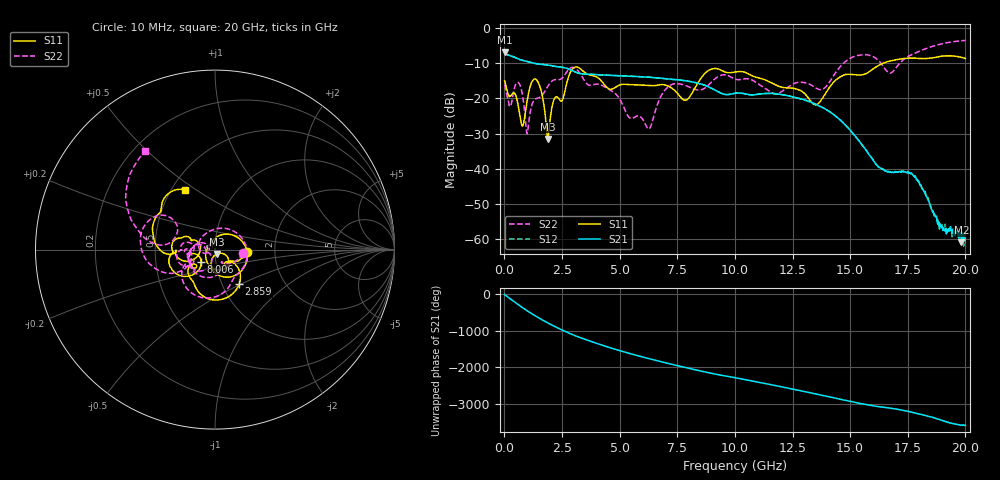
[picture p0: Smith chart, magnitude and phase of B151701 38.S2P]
!  2-Port S-parameters saved by WinCal
! VAR MeasName=S-Parameters (CALIBRATED_DATA) read from VNA (N5244A)
! VAR MeasDate=2015-12-24 19:13:49
! VAR NAME=B151701 38
! VAR FILENAME=B151701 38.S2P
! VAR DATE=2015-12-24 19:13:49
! VAR PHYS_PORTS=1,3
# Hz S DB R 50
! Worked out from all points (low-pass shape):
!   801 points, 10 MHz to 20 GHz, reference 50 ohm
!   highest |S21| = -6.86 dB at 10 MHz (marker M1); lowest = -61.0 dB at 19.83 GHz (marker M2)
!   |S21| within 3 dB of the highest: start of sweep to 1.204 GHz
!   lowest |S11| = -31.5 dB at 1.884 GHz (marker M3), VSWR 1.05, Z = 51 - j2.5 ohm
!   |S11| at or under -10 dB: start of sweep to 16.41 GHz
!   |S22| runs from -30.0 to -3.5 dB; largest |S21 - S12| = 0.0011
!   S11 on the Smith chart (normalised r, x): 10 MHz: 1.43, -0.04; 2.859 GHz: 1.20, -0.49; 8.006 GHz: 0.85, -0.12; 20 GHz: 0.59, +0.45
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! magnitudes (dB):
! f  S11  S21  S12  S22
! 10 MHz  -15.0  -6.9  -6.8  -16.1
! 234.9 MHz  -19.1  -7.8  -7.8  -22.0
! 534.7 MHz  -20.0  -8.5  -8.5  -15.5
! 759.6 MHz  -27.7  -9.1  -9.1  -18.1
! 1.01 GHz  -19.9  -9.5  -9.5  -29.5
! 1.434 GHz  -15.0  -10.1  -10.1  -19.9
! 1.884 GHz  -31.5  -10.5  -10.4  -16.5
! 2.159 GHz  -20.2  -10.8  -10.8  -14.7
! 2.859 GHz  -12.6  -11.8  -11.8  -11.4
! 3.358 GHz  -11.9  -13.0  -13.0  -13.7
! 6.232 GHz  -16.3  -13.9  -13.9  -28.6
! 6.682 GHz  -16.2  -14.2  -14.2  -20.9
! 8.006 GHz  -19.8  -15.1  -15.1  -16.7
! 8.881 GHz  -11.9  -16.8  -16.8  -16.0
! 10.01 GHz  -12.5  -18.5  -18.5  -14.5
! 13.35 GHz  -21.3  -21.2  -21.2  -16.3
! 15.4 GHz  -13.3  -32.3  -32.2  -7.6
! 16.68 GHz  -9.4  -40.9  -40.7  -12.7
! 17.75 GHz  -8.5  -42.0  -42.0  -7.3
! 18.88 GHz  -8.1  -57.2  -55.8  -4.6
! 19.83 GHz  -8.3  -61.0  -59.3  -3.6
! 20 GHz  -8.6  -60.1  -61.3  -3.5
